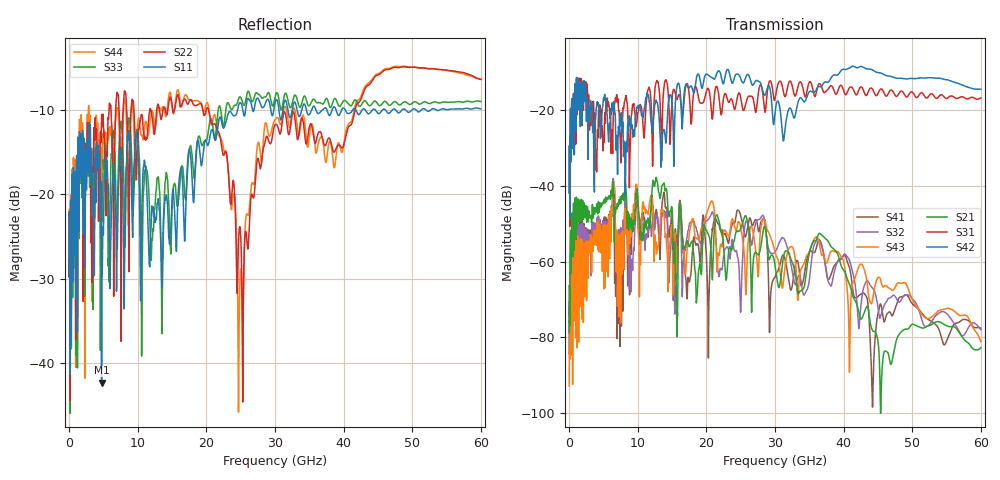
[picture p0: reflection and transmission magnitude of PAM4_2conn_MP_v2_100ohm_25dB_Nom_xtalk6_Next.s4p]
! Info: Touchstone file created by Circ.  Input file=FAB50GbE_2conn_Midplane_Examax_Topo2_v2_100ohm_25dB_Nom.circ
# Hz S RI R 50
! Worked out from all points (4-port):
!   6000 points, 10 MHz to 60 GHz, reference 50 ohm
!   strongest paths, dB at 10 MHz, 15.01 GHz, 30.01 GHz, 45.01 GHz, 60 GHz:
!     S42: -41.7, -18.2, -20.8, -10.2, -14.6
!     S31: -42.0, -17.3, -17.1, -15.7, -16.9
!     S21: -78.8, -46.1, -61.0, -81.0, -82.7
!     S43: -92.8, -51.3, -57.4, -64.2, -81.1
!     S32: -78.4, -52.7, -57.5, -72.1, -78.0
!     S41: -84.2, -47.4, -64.0, -73.7, -77.6
!   lowest |S11| = -42.4 dB at 4.74 GHz (marker M1), VSWR 1.02, Z = 49.3 + j0.318 ohm
!   |S11| at or under -10 dB: start of sweep to 24.55 GHz; 40.23 GHz to 41.32 GHz (1.084 GHz wide, 2.66 % of centre); 43.16 GHz to 44.21 GHz (1.054 GHz wide, 2.41 % of centre)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
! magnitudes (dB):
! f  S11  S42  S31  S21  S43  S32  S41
! 10 MHz  -29.7  -41.7  -42.0  -78.8  -92.8  -78.4  -84.2
! 870 MHz  -17.3  -13.2  -13.3  -43.2  -54.7  -50.4  -49.2
! 4.74 GHz  -42.4  -23.5  -26.1  -44.6  -51.7  -50.2  -51.0
! 20.14 GHz  -14.2  -10.7  -14.5  -52.4  -46.9  -49.2  -65.3
! 24.87 GHz  -9.2  -11.1  -15.8  -51.8  -49.9  -66.8  -47.1
! 28.66 GHz  -9.1  -15.7  -19.6  -51.9  -50.1  -51.9  -51.2
! 60 GHz  -9.9  -14.6  -16.9  -82.7  -81.1  -78.0  -77.6
